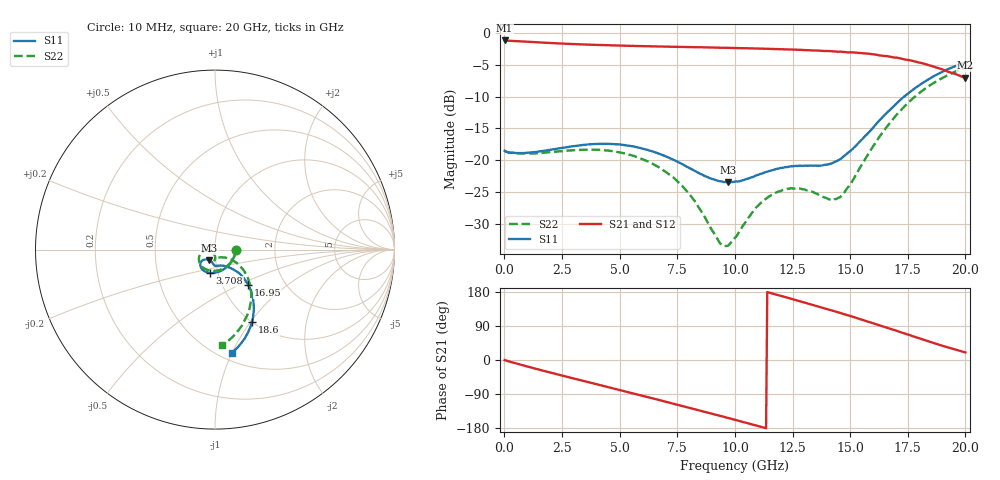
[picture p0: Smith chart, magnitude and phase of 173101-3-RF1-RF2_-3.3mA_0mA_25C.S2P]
!  2-Port S-parameters saved by WinCal
! VAR MeasName=S-Parameters (CALIBRATED_DATA) read from VNA (N5242A)
! VAR MeasDate=2017-7-20 9:34:54
! VAR NAME=173101-3-RF1-RF2_-3.3mA_0mA_25C
! VAR FILENAME=173101-3-RF1-RF2_-3.3mA_0mA_25C.S2P
! VAR DATE=2017-7-20 9:34:54
! VAR PHYS_PORTS=1,2
# Hz S DB R 50
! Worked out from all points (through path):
!   401 points, 10 MHz to 20 GHz, reference 50 ohm
!   highest |S21| = -1.18 dB at 10 MHz (marker M1); lowest = -7.1 dB at 20 GHz (marker M2)
!   group delay of S21, straight-line fit = 46.6 ps
!   lowest |S11| = -23.5 dB at 9.705 GHz (marker M3), VSWR 1.14, Z = 46.6 - j5.51 ohm
!   |S11| at or under -10 dB: start of sweep to 17.34 GHz
!   |S22| runs from -33.5 to -5.4 dB; largest |S21 - S12| = 0.0065
!   S11 on the Smith chart (normalised r, x): 10 MHz: 1.27, -0.00; 3.708 GHz: 0.92, -0.24; 16.95 GHz: 1.32, -0.57; 18.6 GHz: 1.00, -1.02; 20 GHz: 0.57, -1.00
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1e7  -18.53 -0.9  -1.18 -0.2  -1.18 -0.2  -18.50 -1.0
1.50925e9  -18.64 -54.3  -1.49 -25.5  -1.49 -25.5  -18.89 -56.7
3.358325e9  -17.64 -96.0  -1.80 -54.2  -1.80 -54.2  -18.36 -104.6
3.70815e9  -17.50 -101.8  -1.84 -59.5  -1.84 -59.5  -18.35 -111.8
5.10745e9  -17.59 -121.6  -2.00 -80.9  -2.01 -80.9  -18.86 -137.8
6.70665e9  -18.98 -136.4  -2.12 -105.6  -2.12 -105.4  -21.12 -161.6
7.8061e9  -20.83 -139.2  -2.21 -122.6  -2.22 -122.5  -24.42 -172.6
9.355325e9  -23.32 -124.0  -2.32 -147.4  -2.31 -147.3  -33.08 -145.9
9.70515e9  -23.51 -118.2  -2.34 -152.9  -2.33 -152.9  -33.44 -123.3
1.0005e10  -23.38 -113.0  -2.37 -157.8  -2.37 -157.8  -32.20 -105.8
1.085458e10  -22.52 -100.6  -2.44 -171.7  -2.45 -171.6  -27.78 -88.2
1.155422e10  -21.64 -95.7  -2.51 176.6  -2.52 176.8  -25.57 -89.0
1.235382e10  -21.02 -91.7  -2.61 163.1  -2.61 163.3  -24.48 -91.8
1.335332e10  -20.84 -84.3  -2.75 145.9  -2.72 146.1  -24.96 -91.0
1.415292e10  -20.55 -70.9  -2.85 131.7  -2.86 131.8  -26.20 -75.1
1.46027e10  -19.76 -61.2  -2.95 123.5  -2.96 123.8  -25.68 -56.1
1.575212e10  -15.85 -46.1  -3.26 101.6  -3.25 101.8  -19.26 -31.5
1.670165e10  -12.17 -45.7  -3.71 83.1  -3.74 83.1  -14.26 -35.5
1.695152e10  -11.30 -46.8  -3.89 78.3  -3.87 78.4  -13.13 -38.4
1.78011e10  -8.72 -54.1  -4.46 61.1  -4.46 61.2  -10.05 -50.1
1.86007e10  -6.85 -63.1  -5.28 45.3  -5.31 45.5  -7.92 -63.0
2e10  -4.67 -80.9  -7.06 19.9  -7.11 20.5  -5.45 -85.9
